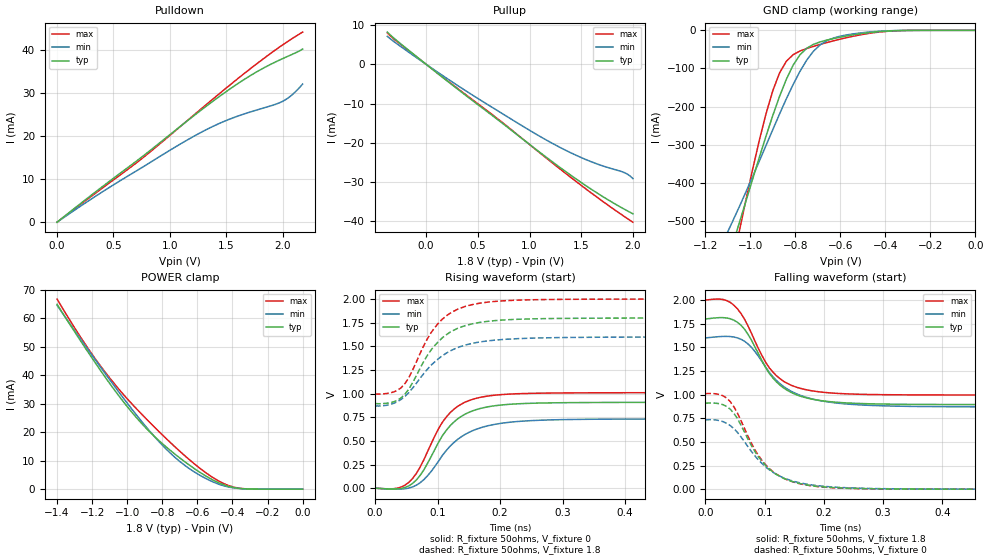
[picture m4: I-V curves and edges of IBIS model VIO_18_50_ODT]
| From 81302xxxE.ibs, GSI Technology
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[Model]   VIO_18_50_ODT
Model_type   I/O
Polarity   Non-Inverting
Vinl  =   0.7000V
Vinh  =   1.1000V
Vmeas =   0.90v
Rref  =   50
|  variable   typ   min   max
C_comp   3.0pF   2.5pF   3.5pF
[Receiver Thresholds]
Vth = 0.90V
Vth_min = 0.80V
Vth_max = 0.95V
Threshold_sensitivity = 1.0
Reference_supply Ext_ref
Vinh_ac = +200mv
Vinh_dc = +100mv
Vinl_ac = -200mv
Vinl_dc = -100mv
Tslew_ac = 550ps
|  variable   typ   min   max
[External Reference]   0.90   0.80   0.95
|  variable   typ   min   max
[Temperature Range]   50   100   0
|  variable   typ   min   max
[Voltage Range]   1.8   1.6   2.0
[Add Submodel]
| Submodel Name   Mode
Weak_ODT_18V   Non-Driving
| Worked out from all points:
|   slope of the pulldown table from 0 to 0.27 V, typ, clamps not added: 48.3 ohm
|   slope of the pullup table from 0 to 0.27 V, typ, clamps not added: 48.1 ohm
|   GND clamp passes 1 mA (typ) near -0.36 V on its own axis
|   POWER clamp passes 1 mA (typ) near -0.42 V on its own axis
|   rising waveform, R_fixture 50ohms, V_fixture 0: 20-80 % time 54.1ps typ, 63.2ps min, 51.5ps max; typ from 0 V to 0.908 V
|   rising waveform, R_fixture 50ohms, V_fixture 1.8: 20-80 % time 56.8ps typ, 66.3ps min, 53.6ps max; typ from 0.894 V to 1.8 V
|   falling waveform, R_fixture 50ohms, V_fixture 1.8: 20-80 % time 57.2ps typ, 67.5ps min, 54.4ps max; typ from 1.8 V to 0.894 V
|   falling waveform, R_fixture 50ohms, V_fixture 0: 20-80 % time 58.4ps typ, 67ps min, 57ps max; typ from 0.908 V to 0 V
[Pullup]
| V(VDDQ-Vout)   typ   min   max
-376mV    8.213mA    7.128mA    8.01mA
-256mV    5.433mA    4.716mA    5.248mA
296mV     -6.144mA   -5.243mA   -5.985mA
680mV     -13.84mA   -11.62mA   -13.63mA
1.088V    -22.17mA   -18.15mA   -22.29mA
1.352V    -27.35mA   -21.91mA   -27.82mA
1.568V    -31.29mA   -24.49mA   -32.17mA
1.904V    -36.69mA   -27.43mA   -38.5mA
1.952V    -37.38mA   -28.04mA   -39.36mA
2V        -38.06mA   -29.09mA   -40.19mA
[PullDown]
| voltage   typ   min   max
0V        -6.731nA   -12.92nA   -7.624nA
352mV     7.255mA    6.21mA     6.966mA
704mV     14.2mA     11.93mA    13.8mA
1.034V    21.04mA    17.25mA    20.92mA
1.276V    26.03mA    20.87mA    26.3mA
1.496V    30.29mA    23.6mA     31.1mA
1.738V    34.45mA    25.82mA    36.17mA
1.98V     37.79mA    27.85mA    40.85mA
2.068V    38.82mA    29.25mA    42.4mA
2.112V    39.34mA    30.27mA    43.14mA
2.178V    40.26mA    32.12mA    44.21mA
[POWER Clamp]
|V(VDDQ-Vout)   typ   min   max
-1.4V     64.83mA    64.49mA    66.68mA
-1.288V   54.1mA     54.59mA    55.43mA
-1.176V   43.77mA    44.87mA    45.19mA
-1.092V   36.42mA    37.75mA    38.39mA
-980mV    27.45mA    28.59mA    30.36mA
-896mV    21.62mA    22.13mA    24.95mA
-812mV    16.64mA    16.22mA    19.79mA
-672mV    9.628mA    8.359mA    11.74mA
-504mV    2.977mA    2.36mA     3.78mA
-392mV    542uA      426.3uA    698.9uA
-308mV    66uA       60.25uA    73.63uA
0V        32.31nA    56.32nA    14.02nA
[GND Clamp]
|(Vout)   typ   min   max
-1.5V     -1.259A    -998.1mA   -1.702A
-1.11V    -621.1mA   -540.5mA   -701.3mA
-1.08V    -564.5mA   -502.7mA   -615.1mA
-1.05V    -506.9mA   -463.9mA   -529.8mA
-930mV    -276.8mA   -301.4mA   -218.1mA
-900mV    -223mA     -260.1mA   -157.9mA
-870mV    -172.8mA   -219.3mA   -111.5mA
-810mV    -91.53mA   -142.2mA   -64mA
-720mV    -36.92mA   -55.09mA   -42.15mA
-630mV    -21.52mA   -20.02mA   -27.43mA
-390mV    -1.864mA   -1.3mA     -2.486mA
0V        -8.791nA   -16.65nA   -9.225nA
[Ramp]
| voltage   typ   min   max
dV/dt_r   0.54/186p   0.48/213p   0.60/209p
dV/dt_f   0.86/129p   0.66/166p   1.07/101p
R_load  =   50ohms
[Rising Waveform]
R_fixture =   50ohms
V_fixture =   0
| Time   V(typ)   V(min)   V(max)
0s        164.1nV    337.9nV    190.4nV
36ps      -7.581mV   -10.38mV   448.1uV
60ps      50.38mV    13.07mV    102.3mV
84ps      263.9mV    131.9mV    387.8mV
102ps     490.5mV    290.5mV    634.8mV
114ps     612.1mV    399mV      752.7mV
132ps     732.8mV    516.2mV    865.3mV
162ps     831mV      623.4mV    950.6mV
264ps     900.3mV    718.6mV    1.005V
600ps     908.2mV    732.9mV    1.01V
[Rising Waveform]
R_fixture =   50ohms
V_fixture =   1.8
V_fixture_min =  1.6
V_fixture_max =  2.0
| Time   V(typ)   V(min)   V(max)
0s        894.4mV    869.7mV    996.1mV
24ps      903.6mV    884.7mV    1.007V
42ps      956.7mV    940.1mV    1.064V
54ps      1.048V     1.011V     1.169V
78ps      1.342V     1.213V     1.508V
96ps      1.512V     1.339V     1.702V
120ps     1.649V     1.451V     1.85V
150ps     1.729V     1.523V     1.933V
252ps     1.791V     1.587V     1.993V
600ps     1.8V       1.6V       2V
[Falling Waveform]
R_fixture =   50ohms
V_fixture =   1.8
V_fixture_min = 1.6
V_fixture_max = 2.0
| Time   V(typ)   V(min)   V(max)
0s        1.8V       1.6V       2V
30ps      1.814V     1.615V     2.006V
54ps      1.766V     1.6V       1.909V
78ps      1.575V     1.499V     1.648V
108ps     1.224V     1.235V     1.284V
132ps     1.071V     1.085V     1.141V
162ps     980.8mV    988.7mV    1.064V
204ps     929.4mV    925.3mV    1.022V
276ps     903.3mV    886.7mV    1.002V
600ps     894.5mV    869.9mV    996.1mV
[Falling Waveform]
R_fixture =   50ohms
V_fixture =   0
| Time   V(typ)   V(min)   V(max)
0s        908.3mV    733.2mV    1.01V
24ps      903.6mV    724.8mV    1.001V
36ps      874.8mV    696.8mV    963.5mV
54ps      749mV      602.2mV    807.7mV
84ps      395.1mV    349.9mV    411.9mV
96ps      292.2mV    269.9mV    300.3mV
120ps     156.4mV    156mV      158.5mV
156ps     64.44mV    72.12mV    62.64mV
264ps     6.326mV    9.722mV    5.038mV
600ps     20.78uV    67.9uV     6.483uV
